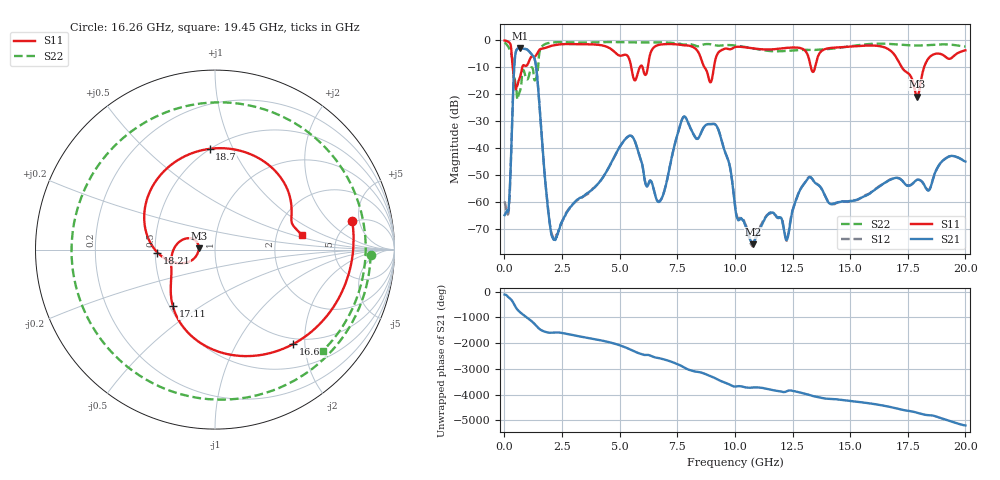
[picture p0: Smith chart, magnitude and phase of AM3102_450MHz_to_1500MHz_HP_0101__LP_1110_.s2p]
!Agilent Technologies,E8364B,MY43040894,A.07.50.67
!Agilent E8364B: A.07.50.67
!Date: Thursday, January 11, 2018 05:43:31
!Correction: S11(Full 2 Port(1,2))
!S21(Full 2 Port(1,2))
!S12(Full 2 Port(1,2))
!S22(Full 2 Port(1,2))
!S2P File: Measurements: S11, S21, S12, S22:
# Hz S  dB  R 50
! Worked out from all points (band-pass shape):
!   1601 points, 10 MHz to 20 GHz, reference 50 ohm
!   highest |S21| = -2.87 dB at 672.2 MHz (marker M1); lowest = -75.6 dB at 10.78 GHz (marker M2)
!   |S21| within 3 dB of the highest: 466.4 MHz to 1.253 GHz (786.4 MHz wide, 91.5 % of centre)
!   lowest |S11| = -20.8 dB at 17.9 GHz (marker M3), VSWR 1.20, Z = 41.7 + j0.63 ohm
!   |S11| at or under -10 dB: 365.2 MHz to 775.9 MHz (410.7 MHz wide, 72 % of centre); 8.68 GHz to 9.09 GHz (410.2 MHz wide, 4.62 % of centre); 17.24 GHz to 18.21 GHz (970.4 MHz wide, 5.48 % of centre)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
!   |S22| runs from -21.9 to -0.7 dB; largest |S21 - S12| = 0.0016
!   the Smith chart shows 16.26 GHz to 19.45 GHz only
!   S11 on the Smith chart (normalised r, x): 16.26 GHz: 4.78, +3.96; 16.66 GHz: 0.89, -1.76; 17.11 GHz: 0.52, -0.39; 18.21 GHz: 0.51, -0.02; 18.7 GHz: 0.50, +0.82; 19.45 GHz: 2.78, +0.59
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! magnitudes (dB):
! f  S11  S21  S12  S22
! 10 MHz  -0.1  -64.8  -59.7  -0.8
! 184.9 MHz  -0.6  -62.3  -63.5  -2.7
! 672.2 MHz  -13.8  -2.9  -2.9  -19.0
! 1.347 GHz  -5.9  -8.2  -8.3  -14.7
! 2.109 GHz  -1.9  -73.2  -73.0  -0.8
! 3.346 GHz  -1.5  -58.2  -58.3  -0.9
! 5.457 GHz  -8.1  -35.3  -35.3  -0.8
! 6.682 GHz  -1.7  -59.9  -59.7  -0.8
! 7.806 GHz  -1.9  -28.3  -28.3  -1.6
! 9.218 GHz  -5.5  -31.9  -31.9  -1.9
! 10.01 GHz  -2.5  -61.5  -61.3  -1.9
! 10.78 GHz  -3.0  -75.6  -75.8  -3.0
! 13.34 GHz  -11.3  -51.2  -51.3  -3.6
! 16.26 GHz  -2.1  -54.2  -54.0  -1.2
! 16.66 GHz  -3.3  -52.0  -51.9  -1.3
! 16.68 GHz  -3.4  -51.9  -51.8  -1.3
! 17.11 GHz  -8.1  -51.1  -51.1  -1.6
! 17.9 GHz  -20.8  -51.7  -51.7  -1.9
! 18.21 GHz  -9.9  -53.6  -53.6  -1.9
! 18.7 GHz  -5.0  -48.7  -48.7  -1.6
! 19.45 GHz  -6.2  -42.9  -42.8  -1.7
! 20 GHz  -3.7  -44.9  -44.9  -2.3
